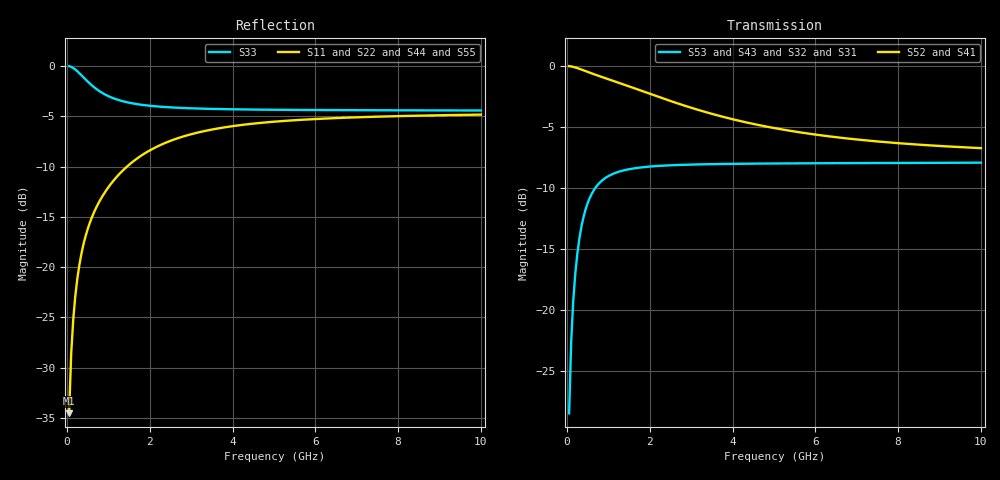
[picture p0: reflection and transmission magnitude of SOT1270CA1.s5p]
! Created Fri Sep 21 14:37:56 2018
# ghz S ma R 50
! 5 Port Network Data from SP1.SP block
! freq  magS11  angS11  magS12  angS12  magS13  angS13  magS14  angS14
!  magS15  angS15
!  magS21  angS21  magS22  angS22  magS23  angS23
!  magS24  angS24  magS25  angS25
!  magS31  angS31  magS32  angS32
!  magS33  angS33  magS34  angS34  magS35  angS35
!  magS41  angS41
!  magS42  angS42  magS43  angS43  magS44  angS44  magS45  angS45
!  magS51  angS51  magS52  angS52  magS53  angS53  magS54  angS54
!  magS55  angS55
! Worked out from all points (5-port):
!   200 points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, 50 MHz to 10 GHz, reference 50 ohm
!   strongest paths, dB at 50 MHz, 2.55 GHz, 5.05 GHz, 7.55 GHz, 10 GHz:
!     S52: 0.0, -2.9, -5.1, -6.2, -6.7
!     S41: 0.0, -2.9, -5.1, -6.2, -6.7
!     S53: -28.5, -8.1, -8.0, -8.0, -7.9
!     S43: -28.5, -8.1, -8.0, -8.0, -7.9
!     S32: -28.5, -8.1, -8.0, -8.0, -8.0
!     S31: -28.5, -8.1, -8.0, -8.0, -8.0
!   lowest |S11| = -34.5 dB at 50 MHz (marker M1), VSWR 1.04, Z = 49.9 - j1.87 ohm
!   |S11| at or under -10 dB: start of sweep to 1.449 GHz
